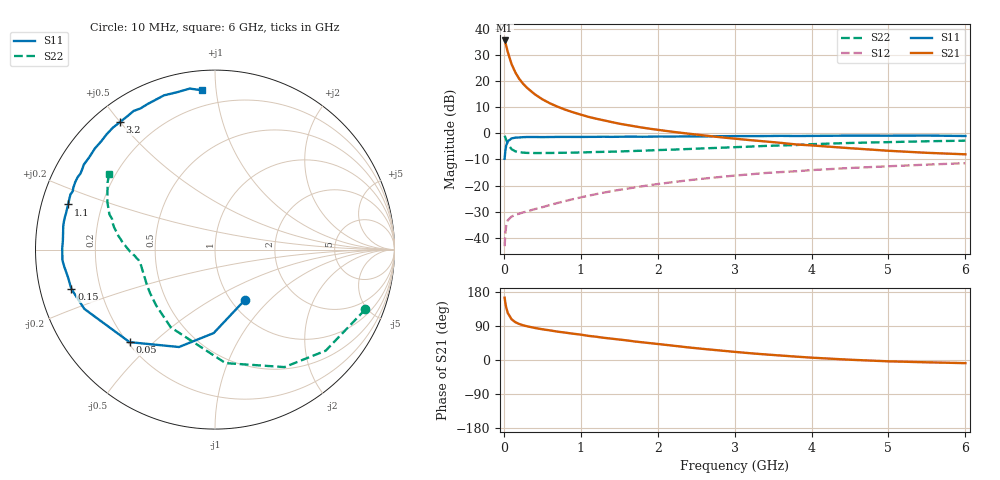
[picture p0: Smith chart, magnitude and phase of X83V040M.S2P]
! SIEMENS Small Signal Semiconductors
! BFP136W
! Si NPN RF Bipolar Junction Transistor in SOT343
! VCE = 3 V  IC = 40 mA
! Common Emitter S-Parameters:  September  1994
# GHz  S  MA  R  50
!  f  S11  S21  S12  S22
! GHz  MAG  ANG  MAG  ANG  MAG  ANG  MAG  ANG
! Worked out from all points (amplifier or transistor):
!   40 points, 10 MHz to 6 GHz, reference 50 ohm
!   highest |S21| = 35.6 dB at 10 MHz (marker M1)
!   |S21| within 3 dB of that: start of sweep to 38.99 MHz
!   unconditionally stable (mu >= 1): 715.1 MHz to 2.799 GHz
!   at 200 MHz: K = 0.49, MSG = 25.8 dB, |S12| = -30.8 dB
!   at 1.5 GHz: K = 1.12, MAG = 10.6 dB, |S12| = -21.6 dB
!   at 6 GHz: K = 0.97, MSG = 1.7 dB, |S12| = -11.4 dB
!   S11 on the Smith chart (normalised r, x): 10 MHz: 1.16, -0.72; 50 MHz: 0.21, -0.42; 150 MHz: 0.09, -0.13; 1.1 GHz: 0.08, +0.15; 3.2 GHz: 0.08, +0.50; 6 GHz: 0.11, +0.92
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0.01  0.3257 -59.0  60.27 164.4  0.0069 73.0  0.9013 -21.7
0.02  0.4651 -90.9  54.32 150.4  0.0124 63.9  0.8352 -42.4
0.03  0.5787 -110.3  48.3 139.5  0.0167 54.4  0.7604 -59.4
0.05  0.7017 -132.7  36.65 124.5  0.0215 40.8  0.6352 -84.7
0.1  0.7995 -155.6  21.3 107.5  0.0255 31.6  0.4984 -119.6
0.15  0.8295 -164.6  14.68 99.7  0.0274 31.0  0.452 -136.5
0.2  0.8341 -169.7  11.07 95.0  0.029 31.1  0.4355 -146.2
0.25  0.8455 -173.6  8.948 91.6  0.0306 33.3  0.4278 -152.5
0.3  0.8522 -176.1  7.495 89.1  0.0319 35.2  0.4226 -156.7
0.4  0.8513 179.6  5.646 84.7  0.0353 39.0  0.4203 -162.1
0.5  0.8491 176.4  4.506 81.1  0.0385 42.6  0.4204 -165.6
0.6  0.851 174.1  3.756 78.1  0.0424 45.3  0.4213 -167.8
0.7  0.8554 171.3  3.237 74.8  0.0464 48.2  0.4233 -169.2
0.9  0.8554 167.4  2.533 69.4  0.0549 51.4  0.428 -171.7
1.1  0.8566 162.9  2.072 63.7  0.0638 53.8  0.435 -173.1
1.5  0.8615 156.3  1.535 54.0  0.0827 55.7  0.4503 -175.8
1.8  0.8611 150.6  1.289 46.7  0.0969 55.2  0.4653 -178.0
2.2  0.8692 143.8  1.07 37.8  0.1164 53.6  0.4886 179.1
3.2  0.8863 126.6  0.742 17.9  0.1641 46.3  0.5578 169.8
4.5  0.9052 108.3  0.52 0.7  0.217 34.6  0.6548 156.3
5.5  0.908 98.9  0.424 -6.1  0.2519 26.6  0.7058 148.0
6  0.8903 94.6  0.397 -8.3  0.2688 22.2  0.7247 144.4
